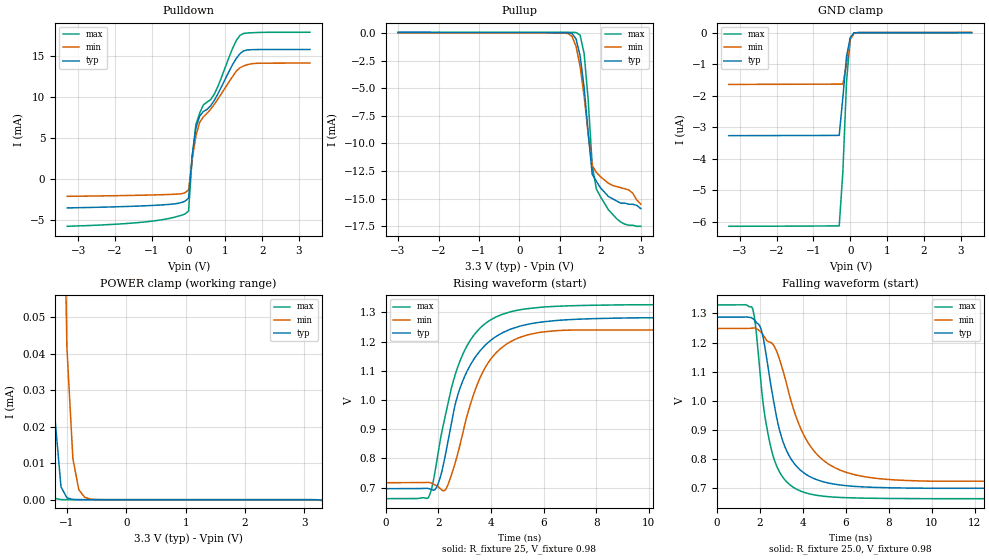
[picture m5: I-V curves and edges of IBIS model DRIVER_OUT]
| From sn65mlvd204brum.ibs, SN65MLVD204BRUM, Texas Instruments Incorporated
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[Model]   DRIVER_OUT
Model_type   3-state
|		 typ	 min	 max
C_comp 5.10247e-12	5.02357e-12	5.17192e-12
Vmeas  = 0.0V
[Temperature Range]		 27.0	 125.0	 -40.0
[Voltage range]		 3.3	 3.0	 3.6
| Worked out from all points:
|   slope of the pulldown table from 0 to 0.495 V, typ, clamps not added: 45.9 ohm
|   POWER clamp passes 1 mA (typ) near -1.46 V on its own axis
|   rising waveform, R_fixture 25, V_fixture 0.98: 20-80 % time 1.28ns typ, 1.2ns min, 1.2ns max; typ from 0.696 V to 1.28 V
|   falling waveform, R_fixture 25.0, V_fixture 0.98: 20-80 % time 1.05ns typ, 1.6ns min, 790ps max; typ from 1.29 V to 0.7 V
[GND_clamp]
|   Voltage   I(typ)   I(min)   I(max)
-3.3V     -3.271uA   -1.644uA   -6.151uA
-300mV    -3.263uA   -1.634uA   -6.138uA
-200mV    -2.051uA   -1.634uA   -4.407uA
-100mV    -747nA     -990.8nA   -1.541uA
0V        -155nA     -220.6nA   -183.5nA
100mV     -6.663nA   -26.08nA   -7.255nA
300mV     -11.24pA   5.787nA    -18.81pA
3.3V      620.2pA    12.61nA    334.5pA
[Power_clamp]
| Note that the[POWER_clamp]voltage table is referenced to Vcc
| and is calculated using Vtable=Vcc - Vmeasured.
|   Voltage   I(typ)   I(min)   I(max)
-1.9V     13.58mA    17.07mA    11.27mA
-1.5V     1.382mA    4.031mA    310.2uA
-1.4V     435.4uA    2.111mA    45.34uA
-1.3V     110.2uA    944.9uA    4.445uA
-1.2V     22.01uA    370.5uA    373.6nA
-1.1V     3.498uA    131.6uA    31.22nA
-1V       511.2nA    41.46uA    3.003nA
-900mV    74.19nA    11.22uA    670.2pA
-800mV    11.4nA     2.742uA    480.8pA
-700mV    2.366nA    650.5nA    456.3pA
-400mV    801pA      19.07nA    401.6pA
3.3V      -155nA     -220.6nA   -183.5nA
[Pulldown]
|   Voltage   I(typ)   I(min)   I(max)
-3.3V     -3.503mA   -2.095mA   -5.743mA
-1.2V     -3.248mA   -1.951mA   -5.217mA
-100mV    -2.692mA   -1.669mA   -4.252mA
0V        -2.327mA   -1.308mA   -3.885mA
100mV     2.911mA    2.418mA    2.786mA
200mV     6.249mA    5.285mA    6.655mA
300mV     7.642mA    6.899mA    8.017mA
400mV     8.224mA    7.56mA     9.022mA
700mV     9.585mA    9.103mA    10.34mA
1.3V      14.7mA     13.16mA    16.88mA
1.6V      15.72mA    13.93mA    17.78mA
3.3V      15.78mA    14.13mA    17.87mA
[Pullup]
|   Voltage   I(typ)   I(min)   I(max)
| Note that the[Pullup]voltage table is referenced to Vcc
| and is calculated using Vtable=Vcc - Vmeasured.
-3V       51.7uA     7.89uA     67.9uA
1.2V      30.8uA     -48.1uA    64.6uA
1.3V      -46.9uA    -303uA     62.6uA
1.4V      -531uA     -1.2mA     49.4uA
1.5V      -2.06mA    -3.03mA    -190uA
1.6V      -4.94mA    -5.74mA    -1.86mA
1.7V      -9.04mA    -9.17mA    -6.05mA
1.8V      -12.8mA    -12mA      -12mA
1.9V      -13.4mA    -12.6mA    -14.1mA
2.4V      -15.2mA    -13.9mA    -16.8mA
2.7V      -15.5mA    -14.2mA    -17.4mA
3V        -15.9mA    -15.5mA    -17.5mA
[Ramp]
|   typ   min   max
dV/dt_r 0.351449/1.28325e-09 0.31383/1.19853e-09 0.398684/1.19531e-09
dV/dt_f 0.352473/7.53198e-10 0.314643/1.05222e-09 0.399146/6.27265e-10
R_load = 25ohm | Note: Measurement is single ended with 25ohm to ground
[Rising Waveform]
R_fixture = 25
V_fixture = 0.98
V_fixture_min = 0.99
V_fixture_max = 0.95
C_fixture = 0p
L_fixture = 0n
|   V(typ)   V(min)   V(max)
0s        696.3mV    716.8mV    662.2mV
1.62ns    696.8mV    718mV      666.4mV
1.93ns    701.7mV    706.6mV    788.6mV
2.26ns    810.4mV    692.3mV    946.1mV
2.87ns    1.053V     865mV      1.145V
3.32ns    1.136V     1.015V     1.219V
3.82ns    1.191V     1.117V     1.265V
5.51ns    1.261V     1.226V     1.314V
9.89ns    1.282V     1.24V      1.327V
9.99us    1.282V     1.24V      1.327V
[Falling Waveform]
R_fixture = 25.0
V_fixture = 0.98
V_fixture_min = 0.99
V_fixture_max = 0.95
C_fixture = 0p
L_fixture = 0n
|   V(typ)   V(min)   V(max)
0s        1.287V     1.248V     1.329V
1.66ns    1.283V     1.25V      1.318V
2.08ns    1.241V     1.234V     1.043V
2.45ns    1.084V     1.202V     862.4mV
2.89ns    908.5mV    1.149V     760mV
3.35ns    813.9mV    1.028V     715mV
4.15ns    747.6mV    868.5mV    683.7mV
5.25ns    716.9mV    780.5mV    670.5mV
9.98ns    699.7mV    724.1mV    664mV
9.99us    699.7mV    724.1mV    664mV
